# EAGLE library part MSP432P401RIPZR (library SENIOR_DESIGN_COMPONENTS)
Low-Power and High Performance 32-Bit ARM Cortex M4F With 256KB Flash and 64KB RAM 100-LQFP -40 to 85
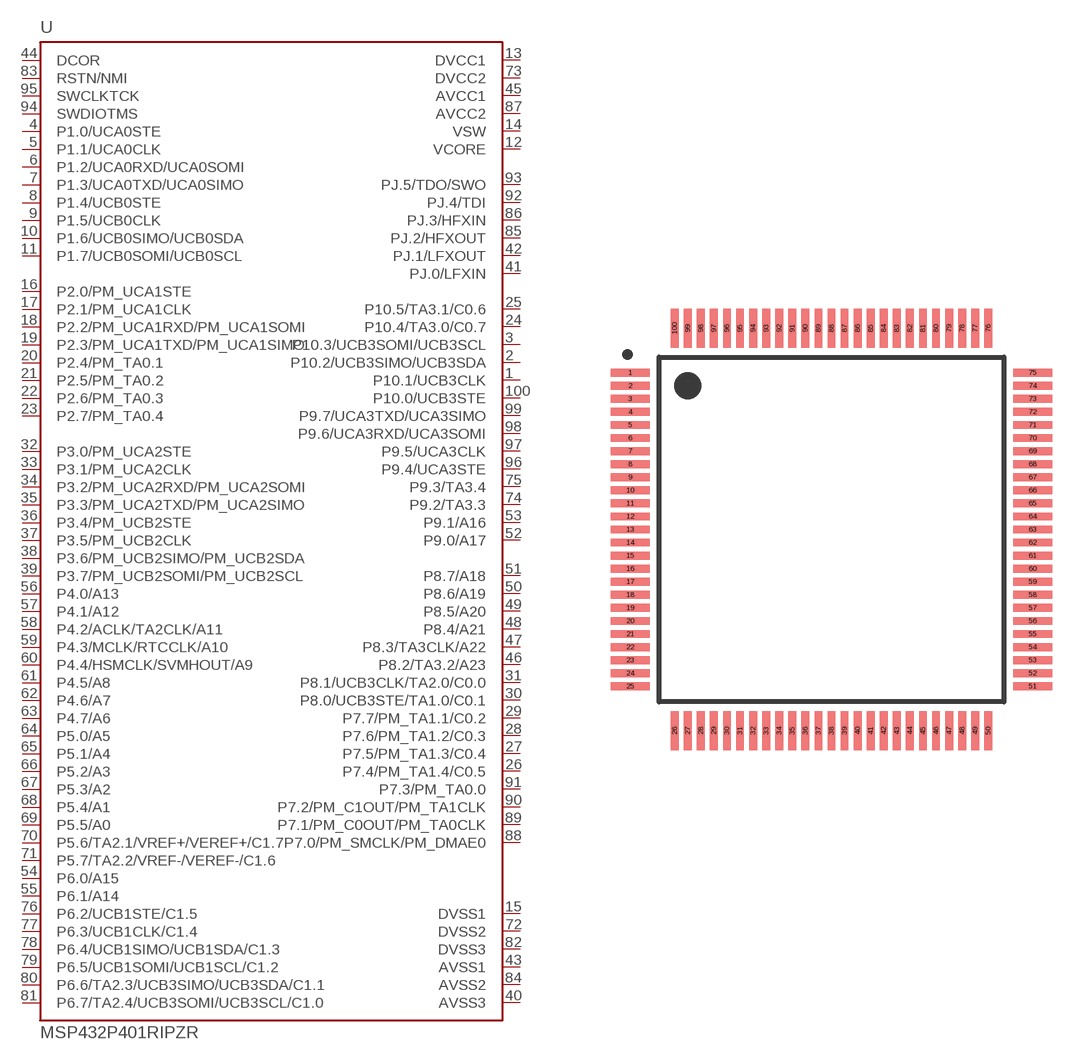
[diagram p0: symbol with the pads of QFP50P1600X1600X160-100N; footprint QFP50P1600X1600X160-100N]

Designator prefix U

## MSP432P401RIPZR (AVAILABILITY: Unavailable; DESCRIPTION: Low-Power and High Performance 32-Bit ARM Cortex M4F With 256KB Flash and 64KB RAM 100-LQFP -40 to 85; MF: Texas Instruments; MP: MSP432P401RIPZR; PACKAGE: LQFP-100 Texas Instruments; PRICE: None)  [QFP50P1600X1600X160-100N]
1  P10.1/UCB3CLK
2  P10.2/UCB3SIMO/UCB3SDA
3  P10.3/UCB3SOMI/UCB3SCL
4  P1.0/UCA0STE
5  P1.1/UCA0CLK
6  P1.2/UCA0RXD/UCA0SOMI
7  P1.3/UCA0TXD/UCA0SIMO
8  P1.4/UCB0STE
9  P1.5/UCB0CLK
10  P1.6/UCB0SIMO/UCB0SDA
11  P1.7/UCB0SOMI/UCB0SCL
12  VCORE  pwr
13  DVCC1  pwr
14  VSW  pwr
15  DVSS1  pwr
16  P2.0/PM_UCA1STE
17  P2.1/PM_UCA1CLK
18  P2.2/PM_UCA1RXD/PM_UCA1SOMI
19  P2.3/PM_UCA1TXD/PM_UCA1SIMO
20  P2.4/PM_TA0.1
21  P2.5/PM_TA0.2
22  P2.6/PM_TA0.3
23  P2.7/PM_TA0.4
24  P10.4/TA3.0/C0.7
25  P10.5/TA3.1/C0.6
26  P7.4/PM_TA1.4/C0.5
27  P7.5/PM_TA1.3/C0.4
28  P7.6/PM_TA1.2/C0.3
29  P7.7/PM_TA1.1/C0.2
30  P8.0/UCB3STE/TA1.0/C0.1
31  P8.1/UCB3CLK/TA2.0/C0.0
32  P3.0/PM_UCA2STE
33  P3.1/PM_UCA2CLK
34  P3.2/PM_UCA2RXD/PM_UCA2SOMI
35  P3.3/PM_UCA2TXD/PM_UCA2SIMO
36  P3.4/PM_UCB2STE
37  P3.5/PM_UCB2CLK
38  P3.6/PM_UCB2SIMO/PM_UCB2SDA
39  P3.7/PM_UCB2SOMI/PM_UCB2SCL
40  AVSS3  pwr
41  PJ.0/LFXIN
42  PJ.1/LFXOUT
43  AVSS1  pwr
44  DCOR  in
45  AVCC1  pwr
46  P8.2/TA3.2/A23
47  P8.3/TA3CLK/A22
48  P8.4/A21
49  P8.5/A20
50  P8.6/A19
51  P8.7/A18
52  P9.0/A17
53  P9.1/A16
54  P6.0/A15
55  P6.1/A14
56  P4.0/A13
57  P4.1/A12
58  P4.2/ACLK/TA2CLK/A11
59  P4.3/MCLK/RTCCLK/A10
60  P4.4/HSMCLK/SVMHOUT/A9
61  P4.5/A8
62  P4.6/A7
63  P4.7/A6
64  P5.0/A5
65  P5.1/A4
66  P5.2/A3
67  P5.3/A2
68  P5.4/A1
69  P5.5/A0
70  P5.6/TA2.1/VREF+/VEREF+/C1.7
71  P5.7/TA2.2/VREF-/VEREF-/C1.6
72  DVSS2  pwr
73  DVCC2  pwr
74  P9.2/TA3.3
75  P9.3/TA3.4
76  P6.2/UCB1STE/C1.5
77  P6.3/UCB1CLK/C1.4
78  P6.4/UCB1SIMO/UCB1SDA/C1.3
79  P6.5/UCB1SOMI/UCB1SCL/C1.2
80  P6.6/TA2.3/UCB3SIMO/UCB3SDA/C1.1
81  P6.7/TA2.4/UCB3SOMI/UCB3SCL/C1.0
82  DVSS3  pwr
83  RSTN/NMI
84  AVSS2  pwr
85  PJ.2/HFXOUT
86  PJ.3/HFXIN
87  AVCC2  pwr
88  P7.0/PM_SMCLK/PM_DMAE0
89  P7.1/PM_C0OUT/PM_TA0CLK
90  P7.2/PM_C1OUT/PM_TA1CLK
91  P7.3/PM_TA0.0
92  PJ.4/TDI
93  PJ.5/TDO/SWO
94  SWDIOTMS
95  SWCLKTCK
96  P9.4/UCA3STE
97  P9.5/UCA3CLK
98  P9.6/UCA3RXD/UCA3SOMI
99  P9.7/UCA3TXD/UCA3SIMO
100  P10.0/UCB3STE

## Footprint QFP50P1600X1600X160-100N (pad centres in mm)
smd 1.5 x 0.3: 1 -7.7,6; 2 -7.7,5.5; 3 -7.7,5; 4 -7.7,4.5; 5 -7.7,4; 6 -7.7,3.5; 7 -7.7,3; 8 -7.7,2.5; 9 -7.7,2; 10 -7.7,1.5; 11 -7.7,1; 12 -7.7,0.5; 13 -7.7,0; 14 -7.7,-0.5; 15 -7.7,-1; 16 -7.7,-1.5; 17 -7.7,-2; 18 -7.7,-2.5; 19 -7.7,-3; 20 -7.7,-3.5; 21 -7.7,-4; 22 -7.7,-4.5; 23 -7.7,-5; 24 -7.7,-5.5; 25 -7.7,-6; 51 7.7,-6; 52 7.7,-5.5; 53 7.7,-5; 54 7.7,-4.5; 55 7.7,-4; 56 7.7,-3.5; 57 7.7,-3; 58 7.7,-2.5; 59 7.7,-2; 60 7.7,-1.5; 61 7.7,-1; 62 7.7,-0.5; 63 7.7,0; 64 7.7,0.5; 65 7.7,1; 66 7.7,1.5; 67 7.7,2; 68 7.7,2.5; 69 7.7,3; 70 7.7,3.5; 71 7.7,4; 72 7.7,4.5; 73 7.7,5; 74 7.7,5.5; 75 7.7,6
smd 0.3 x 1.5: 26 -6,-7.7; 27 -5.5,-7.7; 28 -5,-7.7; 29 -4.5,-7.7; 30 -4,-7.7; 31 -3.5,-7.7; 32 -3,-7.7; 33 -2.5,-7.7; 34 -2,-7.7; 35 -1.5,-7.7; 36 -1,-7.7; 37 -0.5,-7.7; 38 0,-7.7; 39 0.5,-7.7; 40 1,-7.7; 41 1.5,-7.7; 42 2,-7.7; 43 2.5,-7.7; 44 3,-7.7; 45 3.5,-7.7; 46 4,-7.7; 47 4.5,-7.7; 48 5,-7.7; 49 5.5,-7.7; 50 6,-7.7; 76 6,7.7; 77 5.5,7.7; 78 5,7.7; 79 4.5,7.7; 80 4,7.7; 81 3.5,7.7; 82 3,7.7; 83 2.5,7.7; 84 2,7.7; 85 1.5,7.7; 86 1,7.7; 87 0.5,7.7; 88 0,7.7; 89 -0.5,7.7; 90 -1,7.7; 91 -1.5,7.7; 92 -2,7.7; 93 -2.5,7.7; 94 -3,7.7; 95 -3.5,7.7; 96 -4,7.7; 97 -4.5,7.7; 98 -5,7.7; 99 -5.5,7.7; 100 -6,7.7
